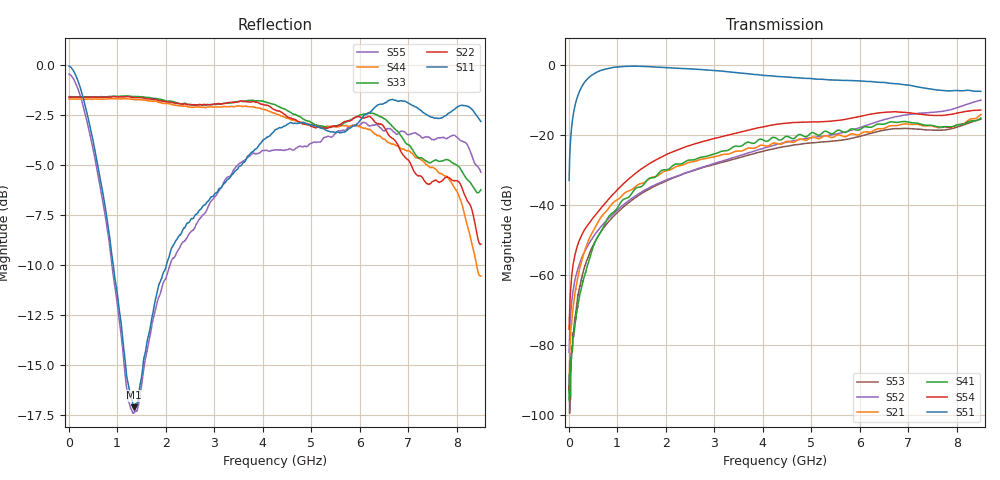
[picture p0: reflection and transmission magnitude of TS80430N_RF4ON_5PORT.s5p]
!Created with skrf (http://scikit-rf.org).
# GHz S RI R 50.0
!freq ReS11 ImS11 ReS12 ImS12 ReS13 ImS13
! ReS14 ImS14 ReS15 ImS15
! ReS21 ImS21 ReS22 ImS22 ReS23 ImS23
! ReS24 ImS24 ReS25 ImS25
! ReS31 ImS31 ReS32 ImS32 ReS33 ImS33
! ReS34 ImS34 ReS35 ImS35
! ReS41 ImS41 ReS42 ImS42 ReS43 ImS43
! ReS44 ImS44 ReS45 ImS45
! ReS51 ImS51 ReS52 ImS52 ReS53 ImS53
! ReS54 ImS54 ReS55 ImS55
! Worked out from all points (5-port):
!   1601 points, 10 MHz to 8.5 GHz, reference 50 ohm
!   strongest paths, dB at 10 MHz, 2.132 GHz, 4.255 GHz, 6.378 GHz, 8.5 GHz:
!     S51: -33.0, -0.9, -3.2, -4.9, -7.6
!     S54: -75.6, -24.9, -17.1, -13.7, -12.9
!     S41: -95.8, -29.0, -20.8, -16.9, -15.2
!     S21: -92.8, -29.7, -22.3, -18.2, -14.2
!     S52: -82.2, -32.3, -22.9, -16.2, -10.1
!     S53: -93.7, -32.4, -23.9, -19.0, -15.5
!   lowest |S11| = -17.1 dB at 1.342 GHz (marker M1), VSWR 1.32, Z = 38.3 + j4.02 ohm
!   |S11| at or under -10 dB: 919.6 MHz to 2.015 GHz (1.095 GHz wide, 74.7 % of centre)
